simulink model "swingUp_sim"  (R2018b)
settings: Solver=ode4  StartTime=0.0  StopTime=T+Tstb  FixedStep=1e-3  MaxStep=1e-3  RelTol=1e-3  AbsTol=1e-6
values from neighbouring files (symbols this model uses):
  b_0 = (bp_0 + bn_0) / 2    [mainSkript_provedeniSimulaceSwingUp.m]    (also in mainSkript_rovniceSystemu.m = (params.bp_0 + params.bn_0) / 2; mainSkript_overeniRovnic.m = 0; mainSkript_simulaceLQG.m = (bn_0 + bp_0) / 2; mainSkript_LQGexperiment.m = (bn_0 + bp_0) / 2)
  b_1 = params.b_1    [mainSkript_provedeniSimulaceSwingUp.m]    (also in mainSkript_rovniceSystemu.m; mainSkript_overeniRovnic.m; mainSkript_kyvadlaNajednouOdhad.m; mainSkript_simulaceLQG.m)
  b_2 = params.b_2    [mainSkript_provedeniSimulaceSwingUp.m]    (also in mainSkript_rovniceSystemu.m; mainSkript_overeniRovnic.m; mainSkript_kyvadlaNajednouOdhad.m; mainSkript_simulaceLQG.m)
  g = 9.81    [mainSkript_provedeniSimulaceSwingUp.m]    (also in mainSkript_rovniceSystemu.m; mainSkript_overeniRovnic.m; mainSkript_estimaceVozik.m; mainSkript_odhadKyvadlaZvlast.m)
  I_1 = params.I_1    [mainSkript_provedeniSimulaceSwingUp.m]    (also in mainSkript_rovniceSystemu.m; mainSkript_overeniRovnic.m; mainSkript_kyvadlaNajednouOdhad.m; mainSkript_simulaceLQG.m)
  I_2 = params.I_2    [mainSkript_provedeniSimulaceSwingUp.m]    (also in mainSkript_rovniceSystemu.m; mainSkript_overeniRovnic.m; mainSkript_kyvadlaNajednouOdhad.m; mainSkript_simulaceLQG.m)
  K = lqr(sysd, Q_lqr, R_lqr)    [mainSkript_provedeniSimulaceSwingUp.m]    (also in makeFBL.m = [0; -d_2*g*sin(th_1); -d_3*g*sin(th_2)]; mainSkript_simulaceLQG.m = lqr(sysd, Qk, Rk); mainSkript_LQGexperiment.m = lqr(sysd, Q, R); mainSkript_LQGexperiment_integral.m = lqr(sysd, Q, R))
  K1 = [K1(1 : idxL-rez); K1(idxL : idxH); K1(idxH+rez : end)]    [mainSkript_provedeniSimulaceSwingUp.m]
  K2 = [K2(1 : idxL-rez); K2(idxL : idxH); K2(idxH+rez : end)]    [mainSkript_provedeniSimulaceSwingUp.m]
  K3 = [K3(1 : idxL-rez); K3(idxL : idxH); K3(idxH+rez : end)]    [mainSkript_provedeniSimulaceSwingUp.m]
  K4 = [K4(1 : idxL-rez); K4(idxL : idxH); K4(idxH+rez : end)]    [mainSkript_provedeniSimulaceSwingUp.m]
  K5 = [K5(1 : idxL-rez); K5(idxL : idxH); K5(idxH+rez : end)]    [mainSkript_provedeniSimulaceSwingUp.m]
  K6 = [K6(1 : idxL-rez); K6(idxL : idxH); K6(idxH+rez : end)]    [mainSkript_provedeniSimulaceSwingUp.m]
  Ki = [Ki(1 : idxL-rez); Ki(idxL : idxH); Ki(idxH+rez : end)]    [mainSkript_provedeniSimulaceSwingUp.m]
  L_1 = params.L_1    [mainSkript_provedeniSimulaceSwingUp.m]    (also in mainSkript_rovniceSystemu.m; mainSkript_overeniRovnic.m; odhadovane_parametry.m = 0.228; mainSkript_kyvadlaNajednouOdhad.m)
  l_1 = params.l_1    [mainSkript_provedeniSimulaceSwingUp.m]    (also in mainSkript_rovniceSystemu.m; mainSkript_overeniRovnic.m; odhadovane_parametry.m = 0.134; mainSkript_kyvadlaNajednouOdhad.m)
  l_2 = params.l_2    [mainSkript_provedeniSimulaceSwingUp.m]    (also in mainSkript_rovniceSystemu.m; mainSkript_overeniRovnic.m; odhadovane_parametry.m = 0.112; mainSkript_kyvadlaNajednouOdhad.m)
  m_0 = params.m_0    [mainSkript_provedeniSimulaceSwingUp.m]    (also in mainSkript_rovniceSystemu.m; mainSkript_overeniRovnic.m; mainSkript_simulaceLQG.m; mainSkript_LQGexperiment.m)
  m_1 = params.m_1    [mainSkript_provedeniSimulaceSwingUp.m]    (also in mainSkript_rovniceSystemu.m; mainSkript_overeniRovnic.m; mainSkript_kyvadlaNajednouOdhad.m; mainSkript_simulaceLQG.m)
  m_2 = params.m_2    [mainSkript_provedeniSimulaceSwingUp.m]    (also in mainSkript_rovniceSystemu.m; mainSkript_overeniRovnic.m; mainSkript_kyvadlaNajednouOdhad.m; mainSkript_simulaceLQG.m)
  q_0 = [theta0(1) theta1(1) theta2(1) dtheta0(1) dtheta1(1) dtheta2(1)]    [mainSkript_provedeniSimulaceSwingUp.m]    (also in mainSkript_kyvadlaNajednouOdhad.m = cell(1, k); mainSkript_simulaceLQG.m = [0 th1_0 th2_0 0 dth1_0 dth2_0]; mainSkript_LQGexperiment.m = zeros(6,1); mainSkript_LQGexperiment_integral.m = zeros(6,1))
  Q_stab = diag([0.1 6e-3 6e-3 1.2 0.6 0.6])    [mainSkript_provedeniSimulaceSwingUp.m]
  Q_swing = diag([10 10 10 100 100 100])    [mainSkript_provedeniSimulaceSwingUp.m]
  R_stab = diag([0.1 0.5 0.5])    [mainSkript_provedeniSimulaceSwingUp.m]
  R_swing = diag([1 1 1])    [mainSkript_provedeniSimulaceSwingUp.m]
  t_FB = [t_FB(1 : idxL-rez); t_FB(idxL : idxH); t_FB(idxH+rez : end)]    [mainSkript_provedeniSimulaceSwingUp.m]
  Ts = 1e-3    (= 0.001)    [mainSkript_provedeniSimulaceSwingUp.m]    (also in mainSkript_rovniceSystemu.m; mainSkript_simulaceLQG.m; mainSkript_LQGexperiment.m; mainSkript_LQGexperiment_integral.m)
undefined symbols (not defined in the file or in its folder): DiscIntNeverNeededParam
libraries: simulink x5, sharedTrackingLibrary x1
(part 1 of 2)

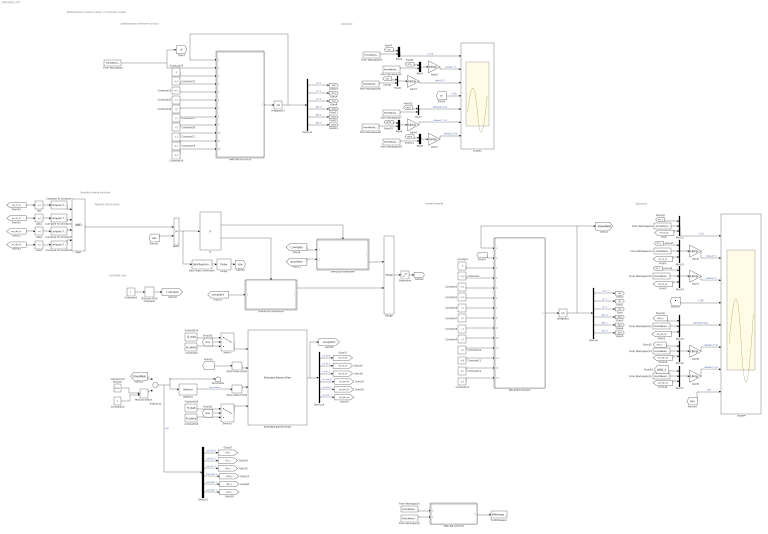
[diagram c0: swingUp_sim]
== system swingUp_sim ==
  note: Simulace realne soustavy
  note: Zjednodusene rovnice (vstup == zrychleni voziku)
  note: Vypocet sily na vozik
  note: pocitadlo casu
  note: Zobrazeni
  note: zobrazeni
  note: model komplet
  note: zjednodusene nelinearni rovnice
  AND : Logic  Inputs=4  AllPortsSameDT=off  OutDataTypeStr=boolean
  AND1 : Logic  Operator=OR  AllPortsSameDT=off  OutDataTypeStr=boolean
  Abs{,1..3} (4 alike) : Abs
  Compare To Constant : simulink/Logic and Bit Operations/Compare To Constant  relop=<=  const=deg2rad(8)  OutDataTypeStr=boolean
  Compare To Constant1 : simulink/Logic and Bit Operations/Compare To Constant  relop=<=  const=deg2rad(8)  OutDataTypeStr=boolean
  Compare To Constant2 : simulink/Logic and Bit Operations/Compare To Constant  relop=<=  const=deg2rad(50)  OutDataTypeStr=boolean
  Compare To Constant3 : simulink/Logic and Bit Operations/Compare To Constant  relop=<=  const=deg2rad(50)  OutDataTypeStr=boolean
  Constant : Constant  Value=g
  Constant1 : Constant  Value=m_0
  Constant10 : Constant  Value=L_1
  Constant11 : Constant  Value=b_0
  Constant12 : Constant  Value=b_1
  Constant13 : Constant  Value=b_2
  Constant14 : Constant  Value=Q_stab  VectorParams1D=off  SampleTime=Ts
  Constant15 : Constant  Commented=on  Value=g
  Constant16 : Constant  Value=R_stab  VectorParams1D=off  SampleTime=Ts
  Constant17 : Constant  Commented=on  Value=L_1
  Constant18 : Constant  Value=R_swing  VectorParams1D=off  SampleTime=Ts
  Constant19 : Constant  Commented=on  Value=b_1
  Constant2 : Constant  Value=m_1
  Constant20 : Constant  Commented=on  Value=b_2
  Constant21 : Constant  Commented=on  Value=m_1
  Constant22 : Constant  Commented=on  Value=m_2
  Constant23 : Constant  Value=0
  Constant25 : Constant  Commented=on  Value=I_1
  Constant26 : Constant  Commented=on  Value=I_2
  Constant27 : Constant  Commented=on  Value=l_1
  Constant28 : Constant  Commented=on  Value=l_2
  Constant3 : Constant  Value=m_2
  Constant4 : Constant
  Constant5 : Constant  Value=Q_swing  VectorParams1D=off  SampleTime=Ts
  Constant6 : Constant  Value=I_1
  Constant7 : Constant  Value=I_2
  Constant8 : Constant  Value=l_1
  Constant9 : Constant  Value=l_2
  Data Type Conversion : DataTypeConversion  OutDataTypeStr=double
  Delay : Delay  DelayLength=1  InitialCondition=0  UseCircularBuffer=on
  Demux : Demux  Outputs=6
  Demux1 : Demux  Commented=on  Outputs=6
  Demux2 : Demux  Outputs=6
  Demux4 : Demux  Outputs=6
  Discrete-Time Integrator : DiscreteIntegrator  SampleTime=1e-3  ICPrevOutput=DiscIntNeverNeededParam  ICPrevScaledInput=DiscIntNeverNeededParam
  Extended Kalman Filter : sharedTrackingLibrary/Extended Kalman Filter  StateTransitionFcn=nonLinKalmFcn  HasStateTransitionJacobianFcn=on  StateTransitionJacobianFcn=countJacobDIP  HasAdditiveProcessNoise=Additive  ProcessNoise=Q_swing  HasTimeVaryingProcessNoise=on  HasStateTransitionFcnExtraArgument=1  InitialState=q_0  InitialStateCovariance=1e-3*eye(6)  MeasurementFcn1=mereniStavuKalm  HasMeasurementJacobianFcn1=off  HasMeasurementEnablePort1=off  HasAdditiveMeasurementNoise1=Additive  MeasurementNoise1=R_swing  HasTimeVaryingMeasurementNoise1=on  HasMeasurementFcnExtraArgument1=0  MeasurementFcn2=myMeasurementFcn  HasMeasurementJacobianFcn2=off  HasMeasurementEnablePort2=off  HasAdditiveMeasurementNoise2=Additive  MeasurementNoise2=1  HasTimeVaryingMeasurementNoise2=off  HasMeasurementFcnExtraArgument2=0  MeasurementFcn3=myMeasurementFcn  HasMeasurementJacobianFcn3=off  HasMeasurementEnablePort3=off  HasAdditiveMeasurementNoise3=Additive  MeasurementNoise3=1  HasTimeVaryingMeasurementNoise3=off  HasMeasurementFcnExtraArgument3=0  MeasurementFcn4=myMeasurementFcn  HasMeasurementJacobianFcn4=off  HasMeasurementEnablePort4=off  HasAdditiveMeasurementNoise4=Additive  MeasurementNoise4=1  HasTimeVaryingMeasurementNoise4=off  HasMeasurementFcnExtraArgument4=0  MeasurementFcn5=myMeasurementFcn  HasMeasurementJacobianFcn5=off  HasMeasurementEnablePort5=off  HasAdditiveMeasurementNoise5=Additive  MeasurementNoise5=1  HasTimeVaryingMeasurementNoise5=off  HasMeasurementFcnExtraArgument5=0  EnableMultirate=off  StateTransitionFcnSampleTime=1  MeasurementFcn1SampleTime=1  MeasurementFcn2SampleTime=1  MeasurementFcn3SampleTime=1  MeasurementFcn4SampleTime=1  MeasurementFcn5SampleTime=1  UseCurrentEstimator=on  OutputStateCovariance=off  DataType=double  SampleTime=1e-3  NumberOfMeasurements=1
  From Workspace : FromWorkspace  Commented=on  VariableName=u_str  SampleTime=0
  From Workspace1 : FromWorkspace  VariableName=ref_traj  SampleTime=0
  From Workspace11 : FromWorkspace  VariableName=theta1_str  SampleTime=0
  From Workspace12 : FromWorkspace  VariableName=theta2_str  SampleTime=0
  From Workspace13 : FromWorkspace  VariableName=dtheta0_str  SampleTime=0
  From Workspace14 : FromWorkspace  VariableName=dtheta1_str  SampleTime=0
  From Workspace15 : FromWorkspace  VariableName=dtheta2_str  SampleTime=0
  From Workspace2 : FromWorkspace  VariableName=u_str  SampleTime=0
  From Workspace3 : FromWorkspace  VariableName=theta0_str  SampleTime=0
  From Workspace4 : FromWorkspace  Commented=on  VariableName=theta0_str  SampleTime=0
  From Workspace5 : FromWorkspace  Commented=on  VariableName=theta1_str  SampleTime=0
  From Workspace6 : FromWorkspace  Commented=on  VariableName=theta2_str  SampleTime=0
  From Workspace7 : FromWorkspace  Commented=on  VariableName=dtheta0_str  SampleTime=0
  From Workspace8 : FromWorkspace  Commented=on  VariableName=dtheta1_str  SampleTime=0
  From Workspace9 : FromWorkspace  Commented=on  VariableName=dtheta2_str  SampleTime=0
  Gain{2..5} (4 alike) : Gain  Commented=on  Gain=180/pi
  Gain{6..9} (4 alike) : Gain  Gain=180/pi
  If : If  IfExpression=u1 == 0
  Integrator : Integrator  InitialCondition=q_0
  Integrator1 : Integrator  Commented=on  InitialCondition=q_0
  MATLAB Function : MATLAB Function  TreatAsAtomicUnit=on
  MATLAB Function2 : MATLAB Function  TreatAsAtomicUnit=on
  MATLAB Function3 : MATLAB Function  Commented=on  TreatAsAtomicUnit=on
  Manual Switch : ManualSwitch
  Merge : Merge
  Mux{11,13..17} (6 alike) : Mux  Inputs=3
  Mux{4..9} (6 alike) : Mux  Commented=on  Inputs=2
  Saturation : Saturate  UpperLimit=50  LowerLimit=-50
  Scope2 : Scope  NumInputPorts=7
  Scope4 : Scope  NumInputPorts=8
  Selector : Selector  InputPortWidth=6  IndexOptions=Index vector (dialog)  Indices=[1:3]  OutputSizes=1
  Subtract1 : Sum  Inputs=+-
  Switch : Switch  Criteria=u2 > Threshold
  Switch1 : Switch  Criteria=u2 > Threshold
  Terminator : Terminator
  To Workspace : ToWorkspace  VariableName=F_str  SaveFormat=Structure With Time  SampleTime=Ts
  Zero-Order Hold1 : ZeroOrderHold  SampleTime=1e-3
  Zero-Order Hold3 : ZeroOrderHold  SampleTime=1e-3
  nepresnosti senzoru : RandomNumber  Mean=zeros(6,1)  Variance=[1e-6 .* ones(6,1)]  SampleTime=1e-3
  stabilizace subsystem : Subsystem  TreatAsAtomicUnit=on
  swing-up subsystem : Subsystem  TreatAsAtomicUnit=on
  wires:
  Constant2/1 -> MATLAB Function2/5(m_1)
  Constant3/1 -> MATLAB Function2/6(m_2)
  MATLAB Function2/1(dx) -> Integrator/1
  Constant6/1 -> MATLAB Function2/7(I_1)
  Demux/3 -> [th2]  "th_2"
  Constant8/1 -> MATLAB Function2/9(l_1)
  Constant9/1 -> MATLAB Function2/10(l_2)
  Constant12/1 -> MATLAB Function2/13(b_1)
  Demux/2 -> [th1]  "th_1"
  Constant7/1 -> MATLAB Function2/8(I_2)
  Constant11/1 -> MATLAB Function2/12(b_0)
  Constant/1 -> MATLAB Function2/3(g)
  Constant10/1 -> MATLAB Function2/11(L_1)
  Constant13/1 -> MATLAB Function2/14(b_2)
  Constant1/1 -> MATLAB Function2/4(m_0)
  Demux/1 -> [th0]  "th_0"
  Demux/4 -> [dth0]  "dth_0"
  Demux/6 -> [dth2]  "dth_2"
  Demux/5 -> [dth1]  "dth_1"
  Constant28/1 -> MATLAB Function3/9(l_2)
  Demux1/1 -> [sth0]  "th_0"
  Constant20/1 -> MATLAB Function3/12(b_2)
  Constant27/1 -> MATLAB Function3/8(l_1)
  Constant17/1 -> MATLAB Function3/10(L_1)
  Constant22/1 -> MATLAB Function3/5(m_2)
  MATLAB Function3/1(dx) -> Integrator1/1
  Demux1/6 -> [sdth2]  "dth_2"
  Demux1/3 -> [sth2]  "th_2"
  Constant25/1 -> MATLAB Function3/6(I_1)
  Demux1/2 -> [sth1]  "th_1"
  Constant15/1 -> MATLAB Function3/3(g)
  Constant19/1 -> MATLAB Function3/11(b_1)
  Constant26/1 -> MATLAB Function3/7(I_2)
  Constant21/1 -> MATLAB Function3/4(m_1)
  Demux1/4 -> [sdth0]  "dth_0"
  Demux1/5 -> [sdth1]  "dth_1"
  From Workspace6/1 -> Mux6/2
  [sth1] -> Mux5/1
  [sth2] -> Mux6/1
  From Workspace4/1 -> Mux4/2
  Mux6/1 -> Gain3/1
  Mux5/1 -> Gain2/1
  [sth0] -> Mux4/1
  From Workspace5/1 -> Mux5/2
  Mux4/1 -> Scope2/1  "x [m]"
  Gain2/1 -> Scope2/2  "theta1 [°]"
  Gain3/1 -> Scope2/3  "theta2 [°]"
  From Workspace7/1 -> Mux7/2
  Mux9/1 -> Gain5/1
  Mux8/1 -> Gain4/1
  [sdth1] -> Mux8/1
  [sdth2] -> Mux9/1
  From Workspace8/1 -> Mux8/2
  From Workspace9/1 -> Mux9/2
  [sdth0] -> Mux7/1
  Mux7/1 -> Scope2/5  "dtheta0 [m/s]"
  [sF] -> Scope2/4  "F [N]"
  Gain4/1 -> Scope2/6  "dtheta1 [°/s]"
  Gain5/1 -> Scope2/7  "dtheta2 [°/s]"
  Integrator1/1 -> MATLAB Function3/1(y), Demux1/1
  Demux4/4 -> [ext_dth_0k]  "lin dth_0"
  Demux4/6 -> [ext_dth_2k]  "lin dth_2"
  Demux4/1 -> [ext_th_0k]  "lin th_0"
  Demux4/2 -> [ext_th_1k]  "lin th_1"
  Demux4/5 -> [ext_dth_1k]  "lin dth_1"
  [F] -> Zero-Order Hold1/1
  Demux4/3 -> [ext_th_2k]  "lin th_2"
  Extended Kalman Filter/1 -> [stavyKalm], Demux4/1
  Zero-Order Hold1/1 -> Extended Kalman Filter/2
  From Workspace/1 -> [sF], MATLAB Function3/2(u)
  Mux14/1 -> Gain7/1
  Mux11/1 -> Scope4/1  "x [m]"
  From Workspace12/1 -> Mux14/2
  [th2_s] -> Mux14/1
  [F] -> Scope4/4  "F [N]"
  Mux15/1 -> Scope4/5  "dtheta0 [m/s]"
  [dth1_s] -> Mux16/1
  Gain6/1 -> Scope4/2  "theta1 [°]"
  [dth0_s] -> Mux15/1
  [th1_s] -> Mux13/1
  [dth2_s] -> Mux17/1
  [th0_s] -> Mux11/1
  Gain8/1 -> Scope4/6  "dtheta1 [°/s]"
  Mux17/1 -> Gain9/1
  From Workspace14/1 -> Mux16/2
  From Workspace15/1 -> Mux17/2
  From Workspace13/1 -> Mux15/2
  From Workspace3/1 -> Mux11/2
  Mux16/1 -> Gain8/1
  Gain7/1 -> Scope4/3  "theta2 [°]"
  From Workspace11/1 -> Mux13/2
  Mux13/1 -> Gain6/1
  Gain9/1 -> Scope4/7  "dtheta2 [°/s]"
  [ext_th_0k] -> Mux11/3
  [ext_th_1k] -> Mux13/3
  [ext_th_2k] -> Mux14/3
  [ext_dth_0k] -> Mux15/3
  [ext_dth_1k] -> Mux16/3
  [ext_dth_2k] -> Mux17/3
  Constant4/1 -> Discrete-Time Integrator/1
  Discrete-Time Integrator/1 -> [t_swingUp]
  Zero-Order Hold3/1 -> Extended Kalman Filter/3
  Subtract1/1 -> Demux2/1, Terminator/1, Selector/1  "vse"
  Integrator/1 -> [stavyReal], MATLAB Function2/1(y), Demux/1
  swing-up subsystem/1(sila na vozik [N]) -> Merge/1
  [F] -> MATLAB Function2/2(u)
  [t_swingUp] -> swing-up subsystem/1(cas Swing-upu [s])
  [stavyKalm] -> swing-up subsystem/2(stavy)
  If/1 -> swing-up subsystem/Action
  If/2 -> stabilizace subsystem/Action
  [stavyKalm] -> stabilizace subsystem/1(stavy)
  stabilizace subsystem/1(sila na vozik [N]) -> Merge/2
  [ext_th_1k] -> Abs/1
  [ext_th_2k] -> Abs1/1
  Compare To Constant/1 -> AND/1
  Compare To Constant1/1 -> AND/2
  [stavyReal] -> Subtract1/1
  From Workspace1/1 -> MATLAB Function/1(y)
  From Workspace2/1 -> MATLAB Function/2(v)
  MATLAB Function/1(u) -> To Workspace/1
  Merge/1 -> Saturation/1
  Selector/1 -> Zero-Order Hold3/1  "jen polohy"
  Saturation/1 -> [F]
  Demux2/1 -> [th0_s]  "sum th_0"
  Demux2/2 -> [th1_s]  "sum th_1"
  Demux2/3 -> [th2_s]  "sum th_2"
  Demux2/4 -> [dth0_s]  "sum dth_0"
  Demux2/5 -> [dth1_s]  "sum dth_1"
  Demux2/6 -> [dth2_s]  "sum dth_2"
  Switch/1 -> Extended Kalman Filter/1
  Constant14/1 -> Switch/1
  Constant5/1 -> Switch/3
  [stav] -> Switch/2
  [stav] -> Switch1/2
  Constant18/1 -> Switch1/3
  Constant16/1 -> Switch1/1
  Switch1/1 -> Extended Kalman Filter/4
  Data Type Conversion/1 -> Delay/1
  Delay/1 -> [stav]
  Manual Switch/1 -> Subtract1/2
  nepresnosti senzoru/1 -> Manual Switch/1
  Constant23/1 -> Manual Switch/2
  [stav] -> Scope4/8  "stav"
  AND/1 -> AND1/1
  AND1/1 -> Data Type Conversion/1, If/1
  [stav] -> AND1/2
  [ext_dth_2k] -> Abs3/1
  Compare To Constant2/1 -> AND/4
  [ext_dth_1k] -> Abs2/1
  Compare To Constant3/1 -> AND/3
  Abs/1 -> Compare To Constant/1
  Abs1/1 -> Compare To Constant1/1
  Abs2/1 -> Compare To Constant3/1
  Abs3/1 -> Compare To Constant2/1

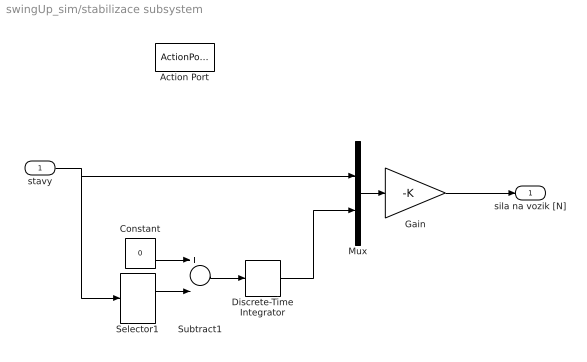
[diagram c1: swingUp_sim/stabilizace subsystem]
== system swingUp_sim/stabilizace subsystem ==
  stavy : Inport
  Action Port : ActionPort  ActionType=else
  Constant : Constant  Value=0
  Discrete-Time Integrator : DiscreteIntegrator  SampleTime=Ts  ICPrevOutput=DiscIntNeverNeededParam  ICPrevScaledInput=DiscIntNeverNeededParam
  Gain : Gain  Gain=-K  Multiplication=Matrix(K*u) (u vector)
  Mux : Mux  Inputs=2
  Selector1 : Selector  InputPortWidth=6  IndexOptions=Index vector (dialog)  Indices=[1]  OutputSizes=1
  Subtract1 : Sum  Inputs=+-
  sila na vozik [N] : Outport
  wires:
  Gain/1 -> sila na vozik [N]/1
  Selector1/1 -> Subtract1/2
  Subtract1/1 -> Discrete-Time Integrator/1
  stavy/1 -> Selector1/1, Mux/1
  Discrete-Time Integrator/1 -> Mux/2
  Constant/1 -> Subtract1/1
  Mux/1 -> Gain/1

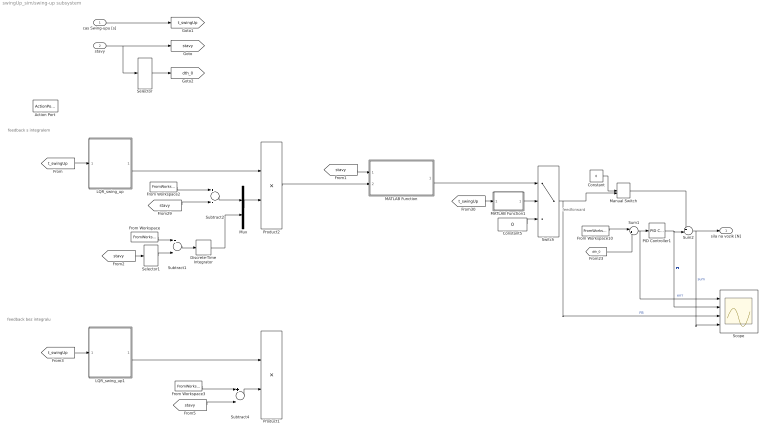
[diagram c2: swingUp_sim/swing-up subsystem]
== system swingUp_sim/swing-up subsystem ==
  note: feedback s integralem
  note: feedforward
  note: feedback bez integralu
  cas Swing-upu [s] : Inport
  stavy : Inport  Port=2
  Action Port : ActionPort  ActionType=then
  Constant : Constant  Value=0
  Constant5 : Constant  Value=0
  Discrete-Time Integrator : DiscreteIntegrator  SampleTime=Ts  ICPrevOutput=DiscIntNeverNeededParam  ICPrevScaledInput=DiscIntNeverNeededParam
  From Workspace : FromWorkspace  VariableName=theta0_str  SampleTime=Ts
  From Workspace10 : FromWorkspace  VariableName=dtheta0_str  SampleTime=1e-3
  From Workspace2 : FromWorkspace  VariableName=ref_traj  SampleTime=1e-3
  From Workspace3 : FromWorkspace  Commented=on  VariableName=ref_traj  SampleTime=1e-3
  LQR_swing_up : Subsystem
  LQR_swing_up1 : Subsystem  Commented=on
  MATLAB Function : MATLAB Function  TreatAsAtomicUnit=on
  MATLAB Function1 : MATLAB Function  TreatAsAtomicUnit=on
  Manual Switch : ManualSwitch  CurrentSetting=0
  Mux : Mux  Inputs=2
  PID Controller1 : simulink/Continuous/PID Controller  Controller=PID  Form=Parallel  TimeDomain=Discrete-time  SampleTime=1e-3  IntegratorMethod=Forward Euler  FilterMethod=Forward Euler  ControllerParametersSource=internal  P=700  I=2.1e3  D=0  UseFilter=on  N=100  TunerSelectOption=Transfer Function Based (PID Tuner App)  InitialConditionSource=internal  InitialConditionForIntegrator=0  InitialConditionForFilter=0  DifferentiatorICPrevScaledInput=0  ExternalReset=none  TrackingMode=off  Kt=1  LimitOutput=off  UpperSaturationLimit=inf  LowerSaturationLimit=-inf  LinearizeAsGain=on  AntiWindupMode=none  Kb=1  POutMin=[]  POutMax=[]  IOutMin=[]  IOutMax=[]  DOutMin=[]  DOutMax=[]  NOutMin=[]  NOutMax=[]  SumOutMin=[]  SumOutMax=[]  SaturationOutMin=[]  SaturationOutMax=[]  PParamMin=[]  PParamMax=[]  IParamMin=[]  IParamMax=[]  DParamMin=[]  DParamMax=[]  NParamMin=[]  NParamMax=[]  KbParamMin=[]  KbParamMax=[]  KtParamMin=[]  KtParamMax=[]  KbOutMin=[]  KbOutMax=[]  KtOutMin=[]  KtOutMax=[]  IntegratorOutMin=[]  IntegratorOutMax=[]  FilterOutMin=[]  FilterOutMax=[]  SumI1OutMin=[]  SumI1OutMax=[]  SumI2OutMin=[]  SumI2OutMax=[]  SumI3OutMin=[]  SumI3OutMax=[]  SumI4OutMin=[]  SumI4OutMax=[]  SumDOutMin=[]  SumDOutMax=[]  DifferentiatorOutMin=[]  DifferentiatorOutMax=[]  FilterDiffOutCoefMin=[]  FilterDiffOutCoefMax=[]  ReciprocalOutMin=[]  ReciprocalOutMax=[]  SumDenOutMin=[]  SumDenOutMax=[]  SumNumOutMin=[]  SumNumOutMax=[]  DivideOutMin=[]  DivideOutMax=[]  IntegratorContinuousStateAttributes=''  IntegratorStateMustResolveToSignalObject=off  IntegratorRTWStateStorageClass=Auto  FilterContinuousStateAttributes=''  FilterStateMustResolveToSignalObject=off  FilterRTWStateStorageClass=Auto  ParallelPVariant=InternalParameters  IdealPVariant=Disabled  IVariant=InternalParameters  DVariant=InternalParameters  IntegratorVariant=Discrete  SatVariant=Disabled  AWVariant=Passthrough  PCopyVariant=Disabled  TRVariant=Disabled  FdbkBlocksVariant=Forward  IdealPFdbkVariant=Disabled  SatFdbkVariant=Disabled  DerivativeFilterVariant=ForwardEulerFilter  NVariant=InternalParameters  NCopyVariant=Disabled  FilterICVariant=InternalICsFilter  IntegratorICVariant=InternalICs  ExternalResetVariant=Disabled  TRSumVariant=Passthrough  SumFdbkVariant=Disabled  SumVariant=Sum_PID
  Product1 : Product  Commented=on  Multiplication=Matrix(*)
  Product2 : Product  Multiplication=Matrix(*)
  Scope : Scope  NumInputPorts=4
  Selector : Selector  InputPortWidth=6  IndexOptions=Index vector (dialog)  Indices=[4]  OutputSizes=1
  Selector1 : Selector  InputPortWidth=6  IndexOptions=Index vector (dialog)  Indices=[1]  OutputSizes=1
  Subtract1 : Sum  Inputs=+-
  Subtract2 : Sum  Inputs=+-
  Subtract4 : Sum  Commented=on  Inputs=+-
  Sum1 : Sum  Inputs=|+-
  Sum2 : Sum  Inputs=++|
  Switch : Switch  Criteria=u2 ~= 0
  sila na vozik [N] : Outport
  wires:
  From Workspace2/1 -> Subtract2/1
  Sum1/1 -> Scope/1, PID Controller1/1  "errr"
  From Workspace10/1 -> Sum1/1
  PID Controller1/1 -> Scope/2, Sum2/2  "FF"
  [stavy] -> Subtract2/2
  Constant5/1 -> Switch/3
  [t_swingUp] -> MATLAB Function1/1(time)
  MATLAB Function1/1(on) -> Switch/2
  [dth_0] -> Sum1/2
  LQR_swing_up/1(K(t)) -> Product2/1
  cas Swing-upu [s]/1 -> [t_swingUp]
  [t_swingUp] -> LQR_swing_up/1(t)
  stavy/1 -> Selector/1, [stavy]
  Selector/1 -> [dth_0]
  Sum2/1 -> Scope/4, sila na vozik [N]/1  "sum"
  Switch/1 -> Scope/3, Manual Switch/2  "FB"
  Manual Switch/1 -> Sum2/1
  Constant/1 -> Manual Switch/1
  MATLAB Function/1(u) -> Switch/1
  [stavy] -> MATLAB Function/1(y)
  Mux/1 -> Product2/2
  Subtract2/1 -> Mux/1
  From Workspace/1 -> Subtract1/1
  Selector1/1 -> Subtract1/2
  [stavy] -> Selector1/1
  Subtract1/1 -> Discrete-Time Integrator/1
  Discrete-Time Integrator/1 -> Mux/2
  LQR_swing_up1/1(K(t)) -> Product1/1
  From Workspace3/1 -> Subtract4/1
  [stavy] -> Subtract4/2
  [t_swingUp] -> LQR_swing_up1/1(t)
  Subtract4/1 -> Product1/2
  Product2/1 -> MATLAB Function/2(v)

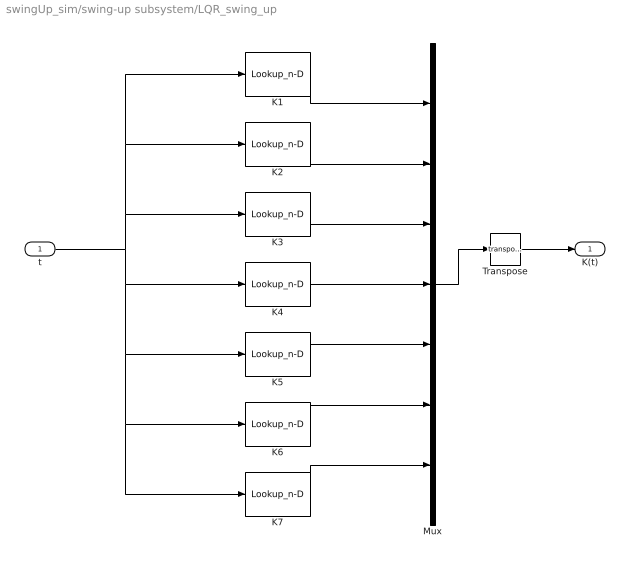
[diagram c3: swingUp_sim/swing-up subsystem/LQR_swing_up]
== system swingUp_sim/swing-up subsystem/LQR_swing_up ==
  t : Inport
  K1 : Lookup_n-D  NumberOfTableDimensions=1  BreakpointsForDimension1=t_FB  Table=K1  InternalRulePriority=Speed  RndMeth=Simplest
  K2 : Lookup_n-D  NumberOfTableDimensions=1  BreakpointsForDimension1=t_FB  Table=K2  InternalRulePriority=Speed  RndMeth=Simplest
  K3 : Lookup_n-D  NumberOfTableDimensions=1  BreakpointsForDimension1=t_FB  Table=K3  InternalRulePriority=Speed  RndMeth=Simplest
  K4 : Lookup_n-D  NumberOfTableDimensions=1  BreakpointsForDimension1=t_FB  Table=K4  InternalRulePriority=Speed  RndMeth=Simplest
  K5 : Lookup_n-D  NumberOfTableDimensions=1  BreakpointsForDimension1=t_FB  Table=K5  InternalRulePriority=Speed  RndMeth=Simplest
  K6 : Lookup_n-D  NumberOfTableDimensions=1  BreakpointsForDimension1=t_FB  Table=K6  InternalRulePriority=Speed  RndMeth=Simplest
  K7 : Lookup_n-D  NumberOfTableDimensions=1  BreakpointsForDimension1=t_FB  Table=Ki  InternalRulePriority=Speed  RndMeth=Simplest
  Mux : Mux  Inputs=7
  Transpose : Math  Operator=transpose
  K(t) : Outport  VectorParamsAs1DForOutWhenUnconnected=on
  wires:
  K5/1 -> Mux/5
  K1/1 -> Mux/1
  K2/1 -> Mux/2
  K6/1 -> Mux/6
  t/1 -> K7/1, K6/1, K5/1, K4/1, K3/1, K2/1, K1/1
  K4/1 -> Mux/4
  K3/1 -> Mux/3
  Mux/1 -> Transpose/1
  Transpose/1 -> K(t)/1
  K7/1 -> Mux/7

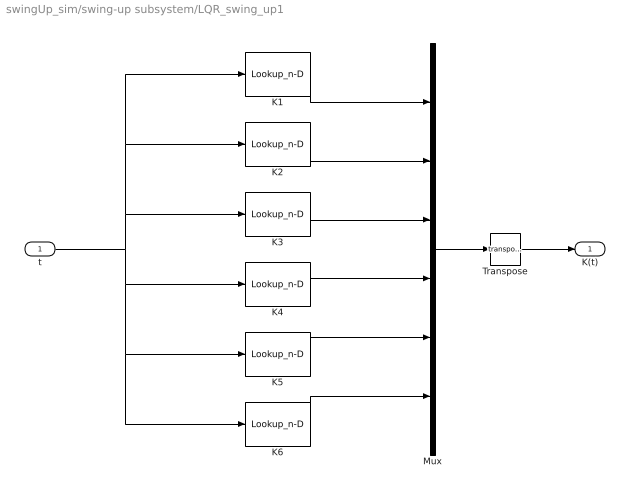
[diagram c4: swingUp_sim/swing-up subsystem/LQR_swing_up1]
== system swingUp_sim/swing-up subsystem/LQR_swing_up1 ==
  t : Inport
  K1 : Lookup_n-D  NumberOfTableDimensions=1  BreakpointsForDimension1=t_FB  Table=K1  InternalRulePriority=Speed  RndMeth=Simplest
  K2 : Lookup_n-D  NumberOfTableDimensions=1  BreakpointsForDimension1=t_FB  Table=K2  InternalRulePriority=Speed  RndMeth=Simplest
  K3 : Lookup_n-D  NumberOfTableDimensions=1  BreakpointsForDimension1=t_FB  Table=K3  InternalRulePriority=Speed  RndMeth=Simplest
  K4 : Lookup_n-D  NumberOfTableDimensions=1  BreakpointsForDimension1=t_FB  Table=K4  InternalRulePriority=Speed  RndMeth=Simplest
  K5 : Lookup_n-D  NumberOfTableDimensions=1  BreakpointsForDimension1=t_FB  Table=K5  InternalRulePriority=Speed  RndMeth=Simplest
  K6 : Lookup_n-D  NumberOfTableDimensions=1  BreakpointsForDimension1=t_FB  Table=K6  InternalRulePriority=Speed  RndMeth=Simplest
  Mux : Mux  Inputs=6
  Transpose : Math  Operator=transpose
  K(t) : Outport  VectorParamsAs1DForOutWhenUnconnected=on
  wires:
  K5/1 -> Mux/5
  K1/1 -> Mux/1
  K2/1 -> Mux/2
  K6/1 -> Mux/6
  K4/1 -> Mux/4
  K3/1 -> Mux/3
  Mux/1 -> Transpose/1
  Transpose/1 -> K(t)/1
  t/1 -> K6/1, K5/1, K4/1, K3/1, K2/1, K1/1

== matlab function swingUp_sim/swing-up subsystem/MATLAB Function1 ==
function on = feedbackOn(time)

on = 0;

if (time <= 0.70)  || (time >= 1.09)
    on = 1;
end

%

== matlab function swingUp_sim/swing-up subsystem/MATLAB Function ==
function u = feedbackLinearization(y, v)
%feedbackLinearization: castecna feedback linearizace - ziskani vstupu pro nelinearni system 

u = (407227096910748504076914119243960960953492563523831375978747126050092199441462516336971030531937534480482304000000*sin(2*y(3)) - 11500407088910324146229444568754977472486398737404017444437732424056822108965631195323726200028988324684156570173440*sin(2*y(2)) - 26418000604491414037729084897799230433872258733859352182489594880568277844574960151329460006886992568489370189824000*v - 45442648452744689114087013101735997253337092110543620748139567159365655238836645966204741088097565259123916800000000*y(4) + 1172314687962316426730830231269620537460387231131907996374896271565425291433805422561032232418857117704806989824000*v*cos(2*y(2)) - 41511426800280173708146189525378283481497712897434391027395221819581263959374364560343632062378953565798400000000*v*cos(2*y(3)) + 492045723340722615495028011226454017452946366853739292052179612616638111902587083211769291479153157578833218567541*y(5)^2*sin(y(2)) + 50295857773834799189479864038880676635514908862422130557322253979452276518744379794851283378667411165394501632000*y(6)^2*sin(y(3)) + 5356276663601442609699708077417056239453993665034575770751736002464515867882739888144337237499995121254400000000000*v*cos(2*y(2) - 2*y(3)) + 7263050669987173942265987748836687610041066651788929085738879757556545879587283107325219312762880000000000000000*cos(2*y(2) - y(3))*y(5) + 9559365284547891329790374180267945472867105459286073908740739843904465123392346919809049805455360000000000000000000*cos(2*y(2) - 2*y(3))*y(4) - 7263050669987173942265987748836687610041066651788929085738879757556545879587283107325219312762880000000000000000*cos(2*y(2) - y(3))*y(6) + 9598375883327782360522300495416211152969762948065962014481980256228086771971518560933848655035928202444800000000*sin(y(2) - 2*y(3))*y(5)^2 + 22282331604835469067702428897433847264384452559489323601535491529380520538303306109460532984911023308800000000000*y(5)*cos(y(2)) - 6178224845503107713832181816779954459693611170215349909809604911723664888652117385880781865730703360000000000000*y(5)*cos(y(3)) - 9017716265682905405409027352953892971060347895536436742159557775367226695516784382665165340536523980800000000000*y(6)*cos(y(2)) + 6178224845503107713832181816779954459693611170215349909809604911723664888652117385880781865730703360000000000000*y(6)*cos(y(3)) + 64496908227243814717814088608977115510649855854183576524253318118857625462989267473669950699504969770336256000000*y(6)^2*sin(2*y(2) - y(3)) - 4270195300250416688401631268211930494099518640040372875987811061856265168098600038736183951360000000000000000000*cos(y(2) - 2*y(3))*y(5) + 1728158897354997701608804393581124427815894932443086303985916132599091409916404886843173109760000000000000000000*cos(y(2) - 2*y(3))*y(6))/(15845632502852867518708790067200000000*(239006967539396035935973030594274634756909155463627229724502722981906396484375*cos(2*y(2) - 2*y(3)) - 1136174764783351394902810531656107874226455178782169636600620141135272382496583));
